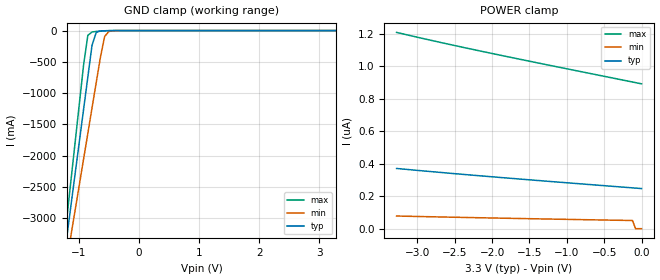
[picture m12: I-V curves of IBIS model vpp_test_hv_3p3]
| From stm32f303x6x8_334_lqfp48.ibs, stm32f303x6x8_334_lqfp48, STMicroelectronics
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|   Model vpp_test_hv_3p3
[Model]  vpp_test_hv_3p3
Model_type Input
Polarity   Non-Inverting
Vinl =   0.990000V
Vinh =   2.310000V
C_comp   2.553700pF   2.511100pF   2.625300pF
[Temperature Range]   25.000000   0.125000k   -40.000000
[Pullup Reference]   3.300000V   2.700000V   3.600000V
[Pulldown Reference]   0.0V   0.0V   0.0V
[POWER Clamp Reference]   3.300000V   2.700000V   3.600000V
[GND Clamp Reference]   0.0V   0.0V   0.0V
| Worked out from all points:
|   GND clamp passes 1 mA (typ) near -0.50 V on its own axis
[GND_clamp]
|Voltage   I(typ)   I(min)   I(max)
-3.3V     -9.956A    -9.78A     -9.768A
-1.27V    -3.813A    -4.083A    -3.618A
-1.2V     -3.301A    -3.676A    -3.004A
-1.13V    -2.789A    -3.269A    -2.389A
-1.06V    -2.278A    -2.863A    -1.774A
-920mV    -1.255A    -2.049A    -545.8mA
-850mV    -743.1mA   -1.642A    -76.56mA
-780mV    -234.4mA   -1.235A    -22.65mA
-710mV    -28.47mA   -828.1mA   -13.73mA
-570mV    -2.673mA   -92.71mA   -4.065mA
-500mV    -982uA     -14.2mA    -1.476mA
3.28V     246.4nA    0A         862nA
[POWER_clamp]
|Voltage   I(typ)   I(min)   I(max)
-3.28V    370.9nA    77.89nA    1.209uA
-2.68V    345.9nA    71.97nA    1.146uA
-2.12V    324nA      66.82nA    1.091uA
-1.4V     297.2nA    60.59nA    1.022uA
-120mV    251.4nA    50.18nA    903.5nA
-80mV     249.9nA    0A         899.8nA
0V        247.1nA    0A         892.3nA
